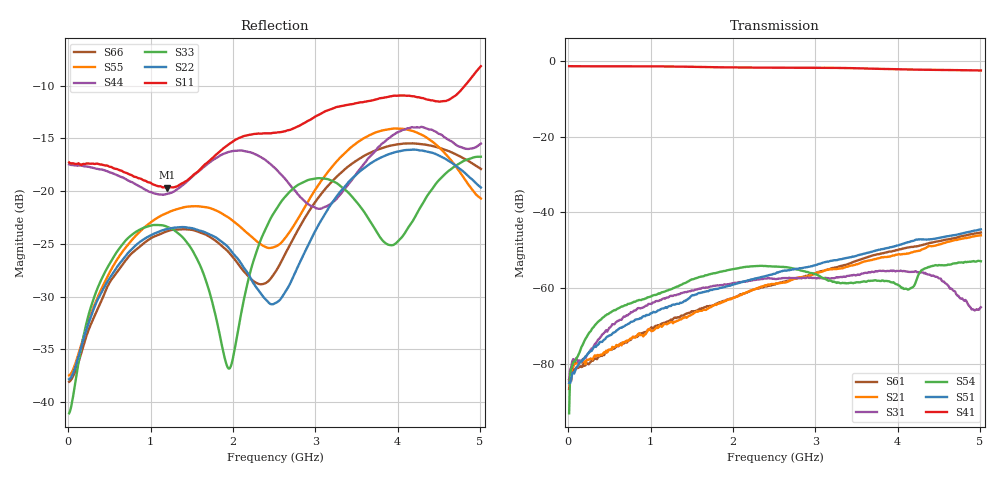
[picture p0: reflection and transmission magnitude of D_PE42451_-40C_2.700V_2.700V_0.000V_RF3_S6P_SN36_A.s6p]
! Device ID: PE42451
! Serial: 36
! Insertion: A
! Temp: -40C
! VDD: 2.700
! Control_Hi: 100.000
! Control_Lo: 0.000
! Logic State: RF3
! Port 1: RFC
! Port 2: RF1
! Port 3: RF2
! Port 4: RF3
! Port 5: RF4
! Port 6: RF5
! V1 = 2.70
! V2 = 2.70
! V3 = 0.00
! V4 = 0.00
! IDD: 1.073120e-05
#  Hz  S  RI  R  50
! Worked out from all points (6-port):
!   401 points, 10 MHz to 5.01 GHz, reference 50 ohm
!   strongest paths, dB at 10 MHz, 1.26 GHz, 2.51 GHz, 3.76 GHz, 5.01 GHz:
!     S41: -1.4, -1.5, -1.8, -2.1, -2.5
!     S51: -85.1, -64.5, -56.2, -50.0, -44.5
!     S54: -93.1, -60.2, -54.4, -58.1, -52.9
!     S31: -84.5, -62.1, -57.6, -55.6, -65.1
!     S21: -86.7, -69.0, -58.9, -52.2, -46.1
!     S61: -84.2, -68.5, -59.1, -51.1, -45.3
!   lowest |S11| = -19.7 dB at 1.198 GHz (marker M1), VSWR 1.23, Z = 55.9 - j9.33 ohm
!   |S11| at or under -10 dB: start of sweep to 4.818 GHz
